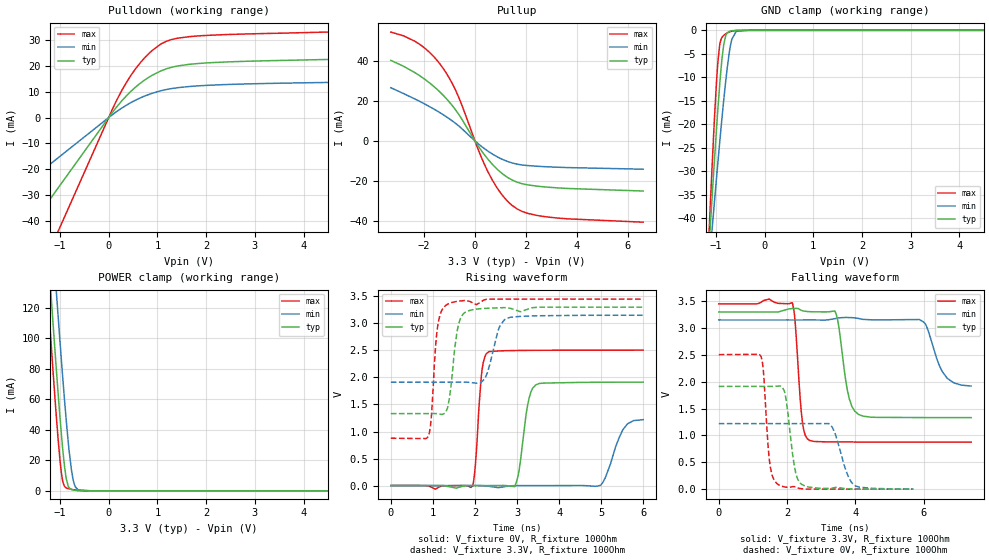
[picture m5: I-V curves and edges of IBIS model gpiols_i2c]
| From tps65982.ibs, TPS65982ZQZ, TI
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|   gpiols_i2c Model
[Model]   gpiols_i2c
Model_type   I/O
Polarity   Non-Inverting
Enable   Active-High
Vinl = 0.80
Vinh = 2.00
Vmeas = 1.65
Vref = 0
Cref = 2pF
Rref = 150
|   typ   min   max
|   (nom PVT)   (fast PVT)   (slow PVT)
C_comp   5.680e-13   5.282e-13   6.367e-13
| Where nom  PVT is Nominal Process, 3.3V, 27C
|   Fast PVT is Strong Process,  3.45V, -40C
|   Slow PVT is Weak Process,   3.15V, 125C
[Voltage Range]   3.3   3.15   3.45
|Junction Temperature
[Temperature Range]   27   125   -40
[Pullup Reference]   3.3   3.15   3.45
[Pulldown Reference]   0   0   0
[Power Clamp Reference]   3.3   3.15   3.45
[GND Clamp Reference]   0   0   0
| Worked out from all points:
|   slope of the pulldown table from 0 to 0.495 V, typ, clamps not added: 45.6 ohm
|   slope of the pullup table from 0 to 0.495 V, typ, clamps not added: 55.2 ohm
|   GND clamp passes 1 mA (typ) near -0.79 V on its own axis
|   POWER clamp passes 1 mA (typ) near -0.77 V on its own axis
|   falling waveform, V_fixture 3.3V, R_fixture 100Ohm: 20-80 % time 265ps typ, 417ps min, 168ps max; typ from 3.3 V to 1.33 V
|   rising waveform, V_fixture 0V, R_fixture 100Ohm: 20-80 % time 196ps typ, 335ps min, 128ps max; typ from 0 V to 1.91 V
|   rising waveform, V_fixture 3.3V, R_fixture 100Ohm: 20-80 % time 178ps typ, 244ps min, 138ps max; typ from 1.33 V to 3.3 V
|   falling waveform, V_fixture 0V, R_fixture 100Ohm: 20-80 % time 228ps typ, 350ps min, 161ps max; typ from 1.91 V to 0 V
[Pulldown]
|   Voltage   I(typ)   I(min)   I(max)
-3.3V     -86.79mA   -49.65mA   -140.2mA
-150.2mV  -3.949mA   -2.259mA   -6.381mA
151.8mV   3.848mA    2.174mA    6.273mA
274.2mV   6.61mA     3.748mA    10.72mA
460.5mV   10.26mA    5.846mA    16.51mA
653.4mV   13.38mA    7.655mA    21.39mA
854.7mV   15.98mA    9.168mA    25.38mA
1.178V    18.86mA    10.85mA    29.54mA
1.422V    20.03mA    11.59mA    30.81mA
2.041V    21.23mA    12.51mA    31.9mA
5.432V    22.9mA     13.9mA     33.63mA
6.6V      23.93mA    14.54mA    35.14mA
[GND Clamp]
|   Voltage   I(typ)   I(min)   I(max)
-3.3V     -444.3mA   -334.2mA   -593.3mA
-1.199V   -56.27mA   -57.44mA   -56.95mA
-1.116V   -42.03mA   -47.13mA   -37.61mA
-1.076V   -35.26mA   -42.18mA   -28.6mA
-988.5mV  -21.26mA   -31.67mA   -11.27mA
-923mV    -11.82mA   -24.06mA   -3.268mA
-838.2mV  -3.019mA   -14.83mA   -1.053mA
-720.1mV  -207.6uA   -4.451mA   -339.4uA
-671.1mV  -87.18uA   -1.876mA   -172.1uA
-581.6mV  -16.64uA   -214uA     -32.75uA
-330mV    -33.38nA   -287.3nA   -22.51nA
6.6V      0A         0A         0A
[Pullup]
|   Voltage   I(typ)   I(min)   I(max)
-3.3V     40.45mA    26.7mA     54.64mA
-2.134V   32.46mA    19.63mA    48.2mA
-1.567V   26.85mA    15.68mA    41.66mA
-1.213V   22.48mA    12.89mA    35.78mA
-626.2mV  13.14mA    7.428mA    21.6mA
146.6mV   -2.904mA   -1.612mA   -4.947mA
521.4mV   -9.378mA   -5.238mA   -15.78mA
1.053V    -16.22mA   -9.118mA   -26.93mA
1.475V    -19.73mA   -11.11mA   -32.55mA
2.005V    -21.92mA   -12.3mA    -36.12mA
2.831V    -23.2mA    -12.99mA   -38.18mA
6.6V      -25.17mA   -14.2mA    -40.81mA
[POWER Clamp]
|   Voltage   I(typ)   I(min)   I(max)
-3.3V     1.18A      1.219A     1.164A
-1.256V   161.6mA    213mA      130.4mA
-1.238V   153.1mA    204.6mA    121.8mA
-1.137V   106.8mA    158.3mA    75.38mA
-1.076V   79.81mA    130.9mA    48.94mA
-970.2mV  36.57mA    84.99mA    11.46mA
-940.2mV  26mA       72.61mA    5.769mA
-871.2mV  7.9mA      45.83mA    1.94mA
-812.5mV  2.002mA    26.11mA    1.349mA
-735.9mV  655.8uA    8.132mA    838.7uA
-625.7mV  235.2uA    675.5uA    309.9uA
6.6V      0A         0A         0A
[Ramp]
R_load = 100
|   typ   min   max
dV/dt_r   1.1482/1.93783e-10   0.732022/3.29942e-10   1.50295/1.2706e-10
dV/dt_f   1.18104/2.62962e-10  0.742596/4.14957e-10   1.54448/1.6615e-10
[Falling Waveform]
V_fixture = 3.3V
V_fixture_min = 3.15V
V_fixture_max = 3.45V
R_fixture = 100Ohm
|   Time   V(typ)   V(min)   V(max)
0s        3.3V       3.15V      3.45V
2.15ns    3.364V     3.15V      3.472V
2.446ns   3.324V     3.15V      1.263V
2.67ns    3.304V     3.15V      905mV
3.406ns   3.306V     3.176V     880.6mV
3.818ns   1.686V     3.195V     878.7mV
4.088ns   1.393V     3.178V     877.8mV
5.986ns   1.333V     3.115V     876.1mV
6.684ns   1.332V     2.065V     876mV
7.384ns   1.332V     1.92V      876mV
[Rising Waveform]
V_fixture = 0V
V_fixture_min = 0V
V_fixture_max = 0V
R_fixture = 100Ohm
|   Time   V(typ)   V(min)   V(max)
0s        2.643nV    40.72nV    1.626nV
1.93ns    -727.5uV   484.1uV    -16.13mV
2.166ns   -342.5uV   -2.132mV   2.129V
2.328ns   -249.4uV   -12.71mV   2.477V
2.95ns    -4.439mV   -330.5uV   2.498V
3.25ns    1.482V     -304.8uV   2.501V
3.446ns   1.864V     -223.1uV   2.502V
4.986ns   1.911V     5.255mV    2.504V
5.514ns   1.912V     1.033V     2.505V
5.998ns   1.914V     1.22V      2.505V
[Rising Waveform]
V_fixture = 3.3V
V_fixture_min = 3.15V
V_fixture_max = 3.45V
R_fixture = 100Ohm
|   Time   V(typ)   V(min)   V(max)
0s        1.331V     1.912V     875.8mV
894ps     1.332V     1.912V     912.6mV
958ps     1.332V     1.912V     1.227V
1.122ns   1.328V     1.912V     2.996V
1.348ns   1.434V     1.912V     3.354V
1.574ns   2.847V     1.912V     3.406V
1.8ns     3.219V     1.912V     3.424V
2.256ns   3.278V     2.013V     3.443V
2.732ns   3.291V     3.084V     3.449V
5.998ns   3.3V       3.15V      3.45V
[Falling Waveform]
V_fixture = 0V
V_fixture_min = 0V
V_fixture_max = 0V
R_fixture = 100Ohm
|   Time   V(typ)   V(min)   V(max)
0s        1.914V     1.22V      2.505V
1.234ns   1.914V     1.22V      2.474V
1.484ns   1.914V     1.22V      530.9mV
1.702ns   1.917V     1.22V      102.4mV
1.922ns   1.824V     1.22V      42.8mV
2.21ns    440.9mV    1.22V      47.39mV
2.43ns    87.75mV    1.22V      7.684mV
3.318ns   17.35mV    1.158V     847.6uV
4.002ns   1.578mV    60.19mV    396uV
5.69ns    217uV      4.325mV    122.2uV
